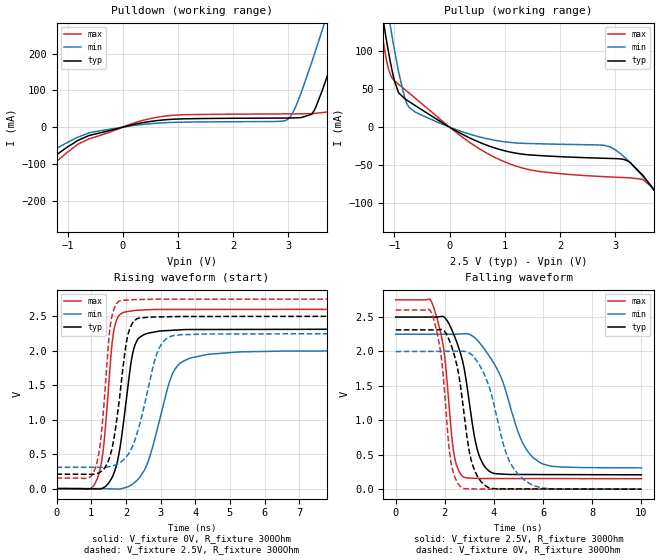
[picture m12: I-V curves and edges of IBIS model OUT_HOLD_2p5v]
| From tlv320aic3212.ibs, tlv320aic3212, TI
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|   OUT_HOLD_2p5v
[Model]   OUT_HOLD_2p5v
Model_type   Output
Polarity   Non-Inverting
Vmeas = 1.25
Vref = 0
Cref = 5pF
Rref = 10000
|   typ   min   max
C_comp   1.444pF   1.430pF   1.479pF
[Voltage Range]   2.5   2.25   2.75
[Temperature Range]   27   125   -40
[Pullup Reference]   2.5   2.25   2.75
[Pulldown Reference]   -0   -0   -0
[Power Clamp Reference]   2.5   2.25   2.75
[GND Clamp Reference]   -0   -0   -0
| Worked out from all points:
|   slope of the pulldown table from 0 to 0.375 V, typ, clamps not added: 30 ohm
|   slope of the pullup table from 0 to 0.375 V, typ, clamps not added: 25.6 ohm
|   falling waveform, V_fixture 2.5V, R_fixture 300Ohm: 20-80 % time 686ps typ, 1.2ns min, 455ps max; typ from 2.5 V to 0.208 V
|   rising waveform, V_fixture 0V, R_fixture 300Ohm: 20-80 % time 372ps typ, 649ps min, 260ps max; typ from 0 V to 2.31 V
|   rising waveform, V_fixture 2.5V, R_fixture 300Ohm: 20-80 % time 356ps typ, 578ps min, 253ps max; typ from 0.208 V to 2.5 V
|   falling waveform, V_fixture 0V, R_fixture 300Ohm: 20-80 % time 592ps typ, 955ps min, 411ps max; typ from 2.31 V to 0 V
[Pulldown]
|   Voltage   I(typ)   I(min)   I(max)
-2.5V     -398.4mA   -334.2mA   -447.4mA
-2.125V   -228.7mA   -175.2mA   -272.4mA
-1.938V   -167.2mA   -129.8mA   -201.8mA
-625mV    -23.69mA   -16.52mA   -32.71mA
762.5mV   19.96mA    12.03mA    30.02mA
2.975V    24.83mA    19.72mA    36.11mA
3.425V    35.1mA     176.6mA    36.98mA
3.612V    98.27mA    262.9mA    39.48mA
3.725V    147.5mA    315.8mA    42.18mA
4.062V    305.3mA    477.1mA    155.4mA
4.138V    341.2mA    513.3mA    190.2mA
4.963V    742.9mA    915.6mA    589.4mA
[Pullup]
|   Voltage   I(typ)   I(min)   I(max)
-2.5V     761.7mA    811.7mA    731.2mA
-1.525V   288.3mA    340.1mA    256.4mA
-1.15V    116.8mA    166.5mA    90.18mA
-1.075V   86.42mA    133.6mA    69.47mA
-925mV    45.42mA    72.92mA    56.55mA
-737.5mV  33.88mA    26.39mA    45.21mA
837.5mV   -27.92mA   -17.56mA   -40.55mA
2.9V      -41.33mA   -25.95mA   -65.74mA
3.237V    -45.09mA   -44.38mA   -66.83mA
3.5V      -63.44mA   -64.76mA   -68.98mA
4.25V     -144.3mA   -139.1mA   -149mA
4.963V    -380.9mA   -433.1mA   -313.3mA
[Ramp]
R_load = 300
|   typ   min   max
dV/dt_r   1.38806/3.70812e-010   1.19923/6.47179e-010   1.56103/2.5971e-010
dV/dt_f   1.37505/6.82386e-010   1.16439/1.19534e-009   1.5587/4.54537e-010
[Falling Waveform]
V_fixture = 2.5V
V_fixture_min = 2.25V
V_fixture_max = 2.75V
R_fixture = 300Ohm
C_fixture = 0F
|   Time   V(typ)   V(min)   V(max)
0s        2.5V       2.25V      2.75V
1.512ns   2.499V     2.25V      2.675V
1.982ns   2.494V     2.25V      1.961V
2.388ns   2.224V     2.249V     480.4mV
2.73ns    1.846V     2.256V     184.9mV
3.32ns    577mV      2.164V     156.8mV
3.811ns   259mV      1.931V     154.4mV
5.067ns   213.2mV    750.9mV    153.9mV
5.621ns   212.6mV    449.6mV    153.7mV
10ns      208.2mV    309.4mV    152.2mV
[Rising Waveform]
V_fixture = 0V
V_fixture_min = 0V
V_fixture_max = 0V
R_fixture = 300Ohm
C_fixture = 0F
|   Time   V(typ)   V(min)   V(max)
0s        809.7nV    2.383uV    240.3nV
1.175ns   -5.414mV   769.7uV    143.6mV
1.368ns   17.52mV    -1.389mV   656.1mV
1.639ns   202.6mV    -5.338mV   2.252V
1.891ns   803.6mV    441.1uV    2.547V
2.162ns   1.871V     54.94mV    2.578V
2.329ns   2.153V     123mV      2.588V
3.333ns   2.297V     1.652V     2.599V
3.761ns   2.308V     1.874V     2.599V
10ns      2.313V     1.999V     2.602V
[Rising Waveform]
V_fixture = 2.5V
V_fixture_min = 2.25V
V_fixture_max = 2.75V
R_fixture = 300Ohm
C_fixture = 0F
|   Time   V(typ)   V(min)   V(max)
0s        208.2mV    309mV      152.2mV
1.112ns   211mV      308.3mV    286.6mV
1.295ns   252.1mV    308.2mV    800.8mV
1.56ns    502.7mV    324mV      2.398V
1.811ns   1.292V     372mV      2.721V
2.006ns   2.097V     457.8mV    2.735V
2.185ns   2.397V     607.6mV    2.741V
2.852ns   2.489V     1.895V     2.748V
3.253ns   2.494V     2.2V       2.748V
10ns      2.5V       2.25V      2.75V
[Falling Waveform]
|Gnd
V_fixture = 0V
V_fixture_min = 0V
V_fixture_max = 0V
R_fixture = 300Ohm
C_fixture = 0F
|   Time   V(typ)   V(min)   V(max)
0s        2.313V     1.999V     2.602V
1.487ns   2.313V     2.001V     2.534V
1.851ns   2.319V     2.001V     1.931V
2.239ns   2.109V     2.002V     414.6mV
2.674ns   1.399V     2.003V     25.59mV
3.029ns   488.2mV    1.968V     4.718mV
3.357ns   168.1mV    1.833V     2.448mV
4.542ns   4.167mV    478.1mV    1.179mV
5.242ns   3.632mV    131.2mV    1.028mV
10ns      3.162uV    157.3uV    133.5nV
